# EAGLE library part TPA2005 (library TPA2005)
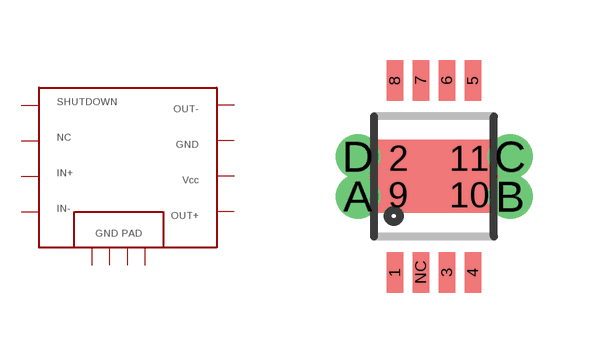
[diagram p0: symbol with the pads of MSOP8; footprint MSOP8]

Designator prefix -

## TPA2005  [MSOP8]
1  P$1
2  P$12
3  P$3  in
4  P$4  in
5  P$5  out
6  P$6
7  P$7
8  P$8  out
9  P$9
10  P$10
11  P$11
A  P$9
B  P$10
C  P$11
D  P$12
NC  P$2  nc

## Footprint MSOP8 (pad centres in mm)
smd 0.41 x 1.02: 1 -0.975,-2.4; 3 0.325,-2.4; 4 0.975,-2.4; 5 0.975,2.4; 6 0.325,2.4; 7 -0.325,2.4; 8 -0.975,2.4; NC -0.325,-2.4
smd 1.778 x 0.914: 2 -0.889,0.457; 9 -0.889,-0.457; 10 0.889,-0.457; 11 0.889,0.457
drill 0.61 pad 1.016: A -1.9,-0.5; B 1.91,-0.5; C 1.91,0.5; D -1.9,0.5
